|   IBIS model for TI xxx DSP
[IBIS Ver]   5.1
[Disclaimer]   Please be aware that in the absence of a written agreement
|   Texas Instruments(TI) assumes no liability for:
|   (1) The accuracy of the IBIS models provided to your company,
|   however, the IBIS model is compliant to industry standard
|   IQ Level 2a.  Refer to IBIS Quality Section below for
|   for full details.
|   (2) The proper functioning of these Models in your design
|   or for any resulting applications
|   (3) Infringement of patents, copyrights or intellectual
|   property rights resulting from your use of these
|   models.
|   TI provides IBIS Models as a service to our customers and
|   therefore reserves the right to limit distribution of the
|   Models.  The information is subject to change without notice.
[File Name]  sprm842a.ibs
[File Rev]   0.3
|   - Initial version
|   - Removed unsupported LVDS models
|   - Removed unsupported IIC and eMMC models
[Date]   19 Oct 2023
[Source]   Texas Instruments Incorporated
[Copyright]   Property of Texas Instruments Incorporated.
|   Unauthorized reproduction and/or distribution is strictly.
|   prohibited.
|   This product is protected under copyright law and trade
|   secret law as an unpublished work.
|   Created 2012,(C) Copyright 1999-2012,
|   Texas Instruments Incorporated., All Rights Reserved.
|   These commodities are under the U.S. Government
|   distribution license control. As such,they are not to be
|   re-exported without the prior approval of the U.S.
|   Department of Commerce.
[Notes]
   This file does not include AMI models for SerDes based links.
   For SerDes simulations use Texas Instruments IBIS AMI models
   Some IV curves contain Non monotonic data points.
|   Revision History
|   GERNERAL COMMENT: All IBIS Quality Notes below reflect latest release
|   and version of IBIS File
|   File passes ibischk5.1 and ibischk6 with 0 errors and 119 warnings
|   Component AM62SiP
[Component] AM62SiP
[Manufacturer] Texas Instruments
[Package]
|   typ   min   max
R_pkg   0.2912   0.11996   0.51217
L_pkg   2.14e-9   9.0745e-10   4.399e-9
C_pkg   6.002e-13   3.435e-13   1.03e-12
[Package Model]   am62sip_pkg
[Pin]	Signal_name	model_name
F6	ATEST0		NC
AE2	ATEST1		NC
AA12	CSI0_ATB_0_H	NC
Y15	CSI0_ATB_1_H	NC
AD15	CSI0_RXCLKN	NC
AE15	CSI0_RXCLKP	NC
AB14	CSI0_RXN0	NC
AD14	CSI0_RXN1	NC
AD13	CSI0_RXN2	NC
AB12	CSI0_RXN3	NC
AC15	CSI0_RXP0	NC
AE14	CSI0_RXP1	NC
AE13	CSI0_RXP2	NC
AC13	CSI0_RXP3	NC
AA14	CSI0_RXRCALIB	NC
R3	DDR_ZQ		NC
T2	DDR0_ATB0	NC
U4	DDR0_ATB1	NC
M2	DDR0_CAL0	NC
G1	DDR0_RESET0_N	NC
E12	EMU0		LVCMOS_V
C11	EMU1		LVCMOS_V
A18	EXT_REFCLK1	LVCMOS_V
D16	EXTINTN		IIC_V
M25	GPMC0_AD0	LVCMOS_H
N23	GPMC0_AD1	LVCMOS_H
T25	GPMC0_AD10	LVCMOS_H
R21	GPMC0_AD11	LVCMOS_H
T22	GPMC0_AD12	LVCMOS_H
T24	GPMC0_AD13	LVCMOS_H
U25	GPMC0_AD14	LVCMOS_H
U24	GPMC0_AD15	LVCMOS_H
N24	GPMC0_AD2	LVCMOS_H
N25	GPMC0_AD3	LVCMOS_H
P24	GPMC0_AD4	LVCMOS_H
P22	GPMC0_AD5	LVCMOS_H
P21	GPMC0_AD6	LVCMOS_H
R23	GPMC0_AD7	LVCMOS_H
R24	GPMC0_AD8	LVCMOS_H
R25	GPMC0_AD9	LVCMOS_H
L23	GPMC0_ADVN_ALE	LVCMOS_H
M24	GPMC0_BE0N_CLE	LVCMOS_H
N20	GPMC0_BE1N	LVCMOS_H
P25	GPMC0_CLK	LVCMOS_H
M21	GPMC0_CSN0	LVCMOS_H
L21	GPMC0_CSN1	LVCMOS_H
K22	GPMC0_CSN2	LVCMOS_H
K24	GPMC0_CSN3	LVCMOS_H
M22	GPMC0_DIR	LVCMOS_H
L24	GPMC0_OEN_REN	LVCMOS_H
U23	GPMC0_WAIT0	LVCMOS_H
V25	GPMC0_WAIT1	LVCMOS_H
L25	GPMC0_WEN	LVCMOS_H
K25	GPMC0_WPN	LVCMOS_H
B16	I2C0_SCL	LVCMOS_V
A16	I2C0_SDA	LVCMOS_V
B17	I2C1_SCL	LVCMOS_V
A17	I2C1_SDA	LVCMOS_V
B1	IFORCE		NC
E15	MCAN0_RX	LVCMOS_V
C15	MCAN0_TX	LVCMOS_V
A20	MCASP0_ACLKR	LVCMOS_V
B20	MCASP0_ACLKX	LVCMOS_V
E19	MCASP0_AFSR	LVCMOS_V
D20	MCASP0_AFSX	LVCMOS_V
E18	MCASP0_AXR0	LVCMOS_V
B18	MCASP0_AXR1	LVCMOS_V
A19	MCASP0_AXR2	LVCMOS_V
B19	MCASP0_AXR3	LVCMOS_V
D1	MCU_ERRORN	LVCMOS_H
A8	MCU_I2C0_SCL	IIC_V
D10	MCU_I2C0_SDA	IIC_V
B3	MCU_MCAN0_RX	LVCMOS_V
D6	MCU_MCAN0_TX	LVCMOS_V
D4	MCU_MCAN1_RX	LVCMOS_V
E5	MCU_MCAN1_TX	LVCMOS_V
B2	MCU_OSC0_XI	NC
A3	MCU_OSC0_XO	NC
D2	MCU_PORZ	RESET_H
B12	MCU_RESETSTATZ	LVCMOS_V
E11	MCU_RESETZ	LVCMOS_V
A7	MCU_SPI0_CLK	LVCMOS_V
E8	MCU_SPI0_CS0	LVCMOS_V
B8	MCU_SPI0_CS1	LVCMOS_V
D9	MCU_SPI0_D0	LVCMOS_V
C9	MCU_SPI0_D1	LVCMOS_V
A6	MCU_UART0_CTSN	LVCMOS_V
B6	MCU_UART0_RTSN	LVCMOS_V
B5	MCU_UART0_RXD	LVCMOS_V
A5	MCU_UART0_TXD	LVCMOS_V
AD24	MDIO0_MDC	LVCMOS_V
AB22	MDIO0_MDIO	LVCMOS_V
AB1	MMC0_CLK	SDIO_H
Y3	MMC0_CMD	SDIO_H
AA2	MMC0_DAT0	SDIO_H
AA1	MMC0_DAT1	SDIO_H
AA3	MMC0_DAT2	SDIO_H
Y4	MMC0_DAT3	SDIO_H
AB2	MMC0_DAT4	SDIO_H
AC1	MMC0_DAT5	SDIO_H
AD2	MMC0_DAT6	SDIO_H
AC2	MMC0_DAT7	SDIO_H
B22	MMC1_CLK	SDIO_V
A21	MMC1_CMD	SDIO_V
A22	MMC1_DAT0	SDIO_V
B21	MMC1_DAT1	SDIO_V
C21	MMC1_DAT2	SDIO_V
D22	MMC1_DAT3	SDIO_V
D17	MMC1_SDCD	LVCMOS_V
C17	MMC1_SDWP	LVCMOS_V
D25	MMC2_CLK	SDIO_H
C24	MMC2_CMD	SDIO_H
B24	MMC2_DAT0	SDIO_H
C25	MMC2_DAT1	SDIO_H
E23	MMC2_DAT2	SDIO_H
D24	MMC2_DAT3	SDIO_H
A23	MMC2_SDCD	LVCMOS_H
B23	MMC2_SDWP	LVCMOS_H
AA5	OLDI0_A0N	LVDS
Y6	OLDI0_A0P	LVDS
AD3	OLDI0_A1N	LVDS
AB4	OLDI0_A1P	LVDS
Y8	OLDI0_A2N	LVDS
AA8	OLDI0_A2P	LVDS
AB6	OLDI0_A3N	LVDS
AA7	OLDI0_A3P	LVDS
AC6	OLDI0_A4N	LVDS
AC5	OLDI0_A4P	LVDS
AE5	OLDI0_A5N	LVDS
AD6	OLDI0_A5P	LVDS
AE6	OLDI0_A6N	LVDS
AD7	OLDI0_A6P	LVDS
AD8	OLDI0_A7N	LVDS
AE7	OLDI0_A7P	LVDS
AD4	OLDI0_CLK0N	LVDS
AE3	OLDI0_CLK0P	LVDS
AE4	OLDI0_CLK1N	LVDS
AD5	OLDI0_CLK1P	LVDS
H24	OSPI0_CLK	LVCMOS_H
F23	OSPI0_CSN0	LVCMOS_H
G21	OSPI0_CSN1	LVCMOS_H
H21	OSPI0_CSN2	LVCMOS_H
E24	OSPI0_CSN3	LVCMOS_H
E25	OSPI0_D0	LVCMOS_H
G24	OSPI0_D1	LVCMOS_H
F25	OSPI0_D2	LVCMOS_H
F24	OSPI0_D3	LVCMOS_H
J23	OSPI0_D4	LVCMOS_H
J25	OSPI0_D5	LVCMOS_H
H25	OSPI0_D6	LVCMOS_H
J22	OSPI0_D7	LVCMOS_H
J24	OSPI0_DQS	LVCMOS_H
G25	OSPI0_LBCLKO	LVCMOS_H
B7	PMIC_LPM_EN0	LVCMOS_V
E21	PORZ_OUT	LVCMOS_V
F20	RESET_REQZ	LVCMOS_V
F22	RESETSTATZ	LVCMOS_V
AB17	RGMII1_RD0	LVCMOS_V
AC17	RGMII1_RD1	LVCMOS_V
AB16	RGMII1_RD2	LVCMOS_V
AA15	RGMII1_RD3	LVCMOS_V
AE17	RGMII1_RX_CTL	LVCMOS_V
AD17	RGMII1_RXC	LVCMOS_V
AE20	RGMII1_TD0	LVCMOS_V
AD20	RGMII1_TD1	LVCMOS_V
AE18	RGMII1_TD2	LVCMOS_V
AD18	RGMII1_TD3	LVCMOS_V
AD19	RGMII1_TX_CTL	LVCMOS_V
AE19	RGMII1_TXC	LVCMOS_V
AE23	RGMII2_RD0	LVCMOS_V
AB20	RGMII2_RD1	LVCMOS_V
AC21	RGMII2_RD2	LVCMOS_V
AE22	RGMII2_RD3	LVCMOS_V
AD22	RGMII2_RX_CTL	LVCMOS_V
AD23	RGMII2_RXC	LVCMOS_V
Y18	RGMII2_TD0	LVCMOS_V
AA18	RGMII2_TD1	LVCMOS_V
AD21	RGMII2_TD2	LVCMOS_V
AC20	RGMII2_TD3	LVCMOS_V
AA19	RGMII2_TX_CTL	LVCMOS_V
AE21	RGMII2_TXC	LVCMOS_V
A14	SPI0_CLK	LVCMOS_V
A13	SPI0_CS0	LVCMOS_V
C13	SPI0_CS1	LVCMOS_V
B13	SPI0_D0		LVCMOS_V
B14	SPI0_D1		LVCMOS_V
A10	TCK		LVCMOS_V
A11	TDI		LVCMOS_V
D12	TDO		LVCMOS_V
E7	TEMP_DIODE_P	NC
B11	TMS		LVCMOS_V
B10	TRSTN		LVCMOS_V
A15	UART0_CTSN	LVCMOS_V
B15	UART0_RTSN	LVCMOS_V
D14	UART0_RXD	LVCMOS_V
E14	UART0_TXD	LVCMOS_V
AE11	USB0_DM		NC
AD11	USB0_DP		NC
C20	USB0_DRVVBUS	LVCMOS_V
AE10	USB0_RCALIB	NC
AC11	USB0_VBUS	NC
AD10	USB1_DM		NC
AE9	USB1_DP		NC
F18	USB1_DRVVBUS	LVCMOS_V
AC9	USB1_RCALIB	NC
AB10	USB1_VBUS	NC
U22	VOUT0_DATA0	LVCMOS_H
V24	VOUT0_DATA1	LVCMOS_H
V20	VOUT0_DATA10	LVCMOS_H
AA23	VOUT0_DATA11	LVCMOS_H
AB25	VOUT0_DATA12	LVCMOS_H
AA24	VOUT0_DATA13	LVCMOS_H
Y22	VOUT0_DATA14	LVCMOS_H
AA21	VOUT0_DATA15	LVCMOS_H
W25	VOUT0_DATA2	LVCMOS_H
W24	VOUT0_DATA3	LVCMOS_H
Y25	VOUT0_DATA4	LVCMOS_H
Y24	VOUT0_DATA5	LVCMOS_H
Y23	VOUT0_DATA6	LVCMOS_H
AA25	VOUT0_DATA7	LVCMOS_H
V21	VOUT0_DATA8	LVCMOS_H
W21	VOUT0_DATA9	LVCMOS_H
Y20	VOUT0_DE	LVCMOS_H
AB24	VOUT0_HSYNC	LVCMOS_H
AC24	VOUT0_PCLK	LVCMOS_H
AC25	VOUT0_VSYNC	LVCMOS_H
A2	VSENSE		NC
A12	WKUP_CLKOUT0	LVCMOS_V
B9	WKUP_I2C0_SCL	IIC_V
A9	WKUP_I2C0_SDA	IIC_V
C2	WKUP_LFOSC0_XI	NC
C1	WKUP_LFOSC0_XO	NC
C6	WKUP_UART0_CTSN	LVCMOS_V
A4	WKUP_UART0_RTSN	LVCMOS_V
B4	WKUP_UART0_RXD	LVCMOS_V
C5	WKUP_UART0_TXD	LVCMOS_V
A1	VSS	GND
A24	VSS	GND
A25	VSS	GND
B25	VSS	GND
E1	VSS	GND
E2	VSS	GND
E3	VSS	GND
F1	VSS	GND
F3	VSS	GND
F4	VSS	GND
F13	VSS	GND
G5	VSS	GND
G13	VSS	GND
G19	VSS	GND
H5	VSS	GND
H6	VSS	GND
H13	VSS	GND
H16	VSS	GND
H18	VSS	GND
H20	VSS	GND
J1	VSS	GND
J2	VSS	GND
J3	VSS	GND
J4	VSS	GND
J7	VSS	GND
J13	VSS	GND
K1	VSS	GND
K2	VSS	GND
K3	VSS	GND
K4	VSS	GND
K7	VSS	GND
K13	VSS	GND
K15	VSS	GND
K19	VSS	GND
L1	VSS	GND
L2	VSS	GND
L5	VSS	GND
L6	VSS	GND
L20	VSS	GND
M1	VSS	GND
M5	VSS	GND
M7	VSS	GND
M8	VSS	GND
M10	VSS	GND
M12	VSS	GND
M13	VSS	GND
M17	VSS	GND
M18	VSS	GND
N6	VSS	GND
N15	VSS	GND
P1	VSS	GND
P4	VSS	GND
P5	VSS	GND
P7	VSS	GND
P10	VSS	GND
P13	VSS	GND
R1	VSS	GND
R5	VSS	GND
R6	VSS	GND
R13	VSS	GND
R15	VSS	GND
R18	VSS	GND
R20	VSS	GND
T1	VSS	GND
T4	VSS	GND
T8	VSS	GND
T13	VSS	GND
T14	VSS	GND
T16	VSS	GND
T17	VSS	GND
T18	VSS	GND
U3	VSS	GND
U8	VSS	GND
U19	VSS	GND
V1	VSS	GND
V5	VSS	GND
V6	VSS	GND
V9	VSS	GND
V10	VSS	GND
V11	VSS	GND
V13	VSS	GND
V16	VSS	GND
V18	VSS	GND
W1	VSS	GND
W5	VSS	GND
W7	VSS	GND
Y1	VSS	GND
Y2	VSS	GND
AA11	VSS	GND
AB9	VSS	GND
AD1	VSS	GND
AD9	VSS	GND
AD12	VSS	GND
AD16	VSS	GND
AD25	VSS	GND
AE1	VSS	GND
AE8	VSS	GND
AE12	VSS	GND
AE16	VSS	GND
AE24	VSS	GND
AE25	VSS	GND
G9	CAP_VDDS_CANUART	POWER
H11	CAP_VDDS_MCU	POWER
H15	CAP_VDDS0	POWER
K18	CAP_VDDS1	POWER
W17	CAP_VDDS2	POWER
P19	CAP_VDDS3	POWER
U7	CAP_VDDS4	POWER
H17	CAP_VDDS5	POWER
J19	CAP_VDDS6	POWER
F8	VDD_CANUART	POWER
H8	VDD_CORE	POWER
J11	VDD_CORE	POWER
J14	VDD_CORE	POWER
K17	VDD_CORE	POWER
L12	VDD_CORE	POWER
L15	VDD_CORE	POWER
M16	VDD_CORE	POWER
N8	VDD_CORE	POWER
N11	VDD_CORE	POWER
N13	VDD_CORE	POWER
P17	VDD_CORE	POWER
R11	VDD_CORE	POWER
R14	VDD_CORE	POWER
U12	VDD_CORE	POWER
V8	VDD_CORE	POWER
V15	VDD_CORE	POWER
V17	VDD_CORE	POWER
W14	VDDA_1P8_CSIRX0	POWER
W9	VDDA_1P8_OLDI0	POWER
W10	VDDA_1P8_OLDI0	POWER
Y11	VDDA_1P8_USB	POWER
Y13	VDDA_3P3_USB	POWER
W13	VDDA_CORE_CSIRX0	POWER
W12	VDDA_CORE_USB	POWER
L11	VDDA_MCU	POWER
U11	VDDA_PLL0	POWER
U15	VDDA_PLL1	POWER
L14	VDDA_PLL2	POWER
T9	VDDA_TEMP0	POWER
G16	VDDA_TEMP1	POWER
J12	VDDR_CORE	POWER
K16	VDDR_CORE	POWER
N12	VDDR_CORE	POWER
N14	VDDR_CORE	POWER
P16	VDDR_CORE	POWER
R12	VDDR_CORE	POWER
T10	VDDR_CORE	POWER
U14	VDDR_CORE	POWER
K9	VDDS_DDR	POWER
L8	VDDS_DDR	POWER
M9	VDDS_DDR	POWER
P9	VDDS_DDR	POWER
R8	VDDS_DDR	POWER
F2	VDDS_DDR_MEM	POWER
G2	VDDS_DDR_MEM	POWER
H1	VDDS_DDR_MEM	POWER
H2	VDDS_DDR_MEM	POWER
N1	VDDS_DDR_MEM	POWER
N2	VDDS_DDR_MEM	POWER
P2	VDDS_DDR_MEM	POWER
R2	VDDS_DDR_MEM	POWER
U1	VDDS_DDR_MEM	POWER
U2	VDDS_DDR_MEM	POWER
V2	VDDS_DDR_MEM	POWER
W2	VDDS_DDR_MEM	POWER
M4	VDDS_MEM_1P8	POWER
N3	VDDS_MEM_1P8	POWER
G7	VDDS_OSC0	POWER
H9	VDDSHV_CANUART	POWER
F11	VDDSHV_MCU	POWER
G12	VDDSHV_MCU	POWER
F15	VDDSHV0		POWER
G14	VDDSHV0		POWER
L18	VDDSHV1		POWER
M19	VDDSHV1		POWER
W16	VDDSHV2		POWER
W19	VDDSHV2		POWER
N18	VDDSHV3		POWER
P18	VDDSHV3		POWER
T19	VDDSHV3		POWER
U18	VDDSHV3		POWER
T7	VDDSHV4		POWER
G17	VDDSHV5		POWER
J18	VDDSHV6		POWER
G10	VMON_1P8_SOC	POWER
K10	VMON_3P3_SOC	POWER
H10	VMON_ER_VSYS	POWER
J8	VPP		POWER
|********************  DIFF PIN  *******************************
[Diff_pin]   inv_pin vdiff tdelay_typ   tdelay_min  tdelay_max
AA5	Y6	NA	NA	NA	NA	||	OLDI0_A0N	&	OLDI0_A0P
AD3	AB4	NA	NA	NA	NA	||	OLDI0_A1N	&	OLDI0_A1P
Y8	AA8	NA	NA	NA	NA	||	OLDI0_A2N	&	OLDI0_A2P
AB6	AA7	NA	NA	NA	NA	||	OLDI0_A3N	&	OLDI0_A3P
AC6	AC5	NA	NA	NA	NA	||	OLDI0_A4N	&	OLDI0_A4P
AE5	AD6	NA	NA	NA	NA	||	OLDI0_A5N	&	OLDI0_A5P
AE6	AD7	NA	NA	NA	NA	||	OLDI0_A6N	&	OLDI0_A6P
AD8	AE7	NA	NA	NA	NA	||	OLDI0_A7N	&	OLDI0_A7P
AD4	AE3	NA	NA	NA	NA	||	OLDI0_CLK0N	&	OLDI0_CLK0P
AE4	AD5	NA	NA	NA	NA	||	OLDI0_CLK1N	&	OLDI0_CLK1P
|****************** SDIO
[Model Selector] SDIO_H
sdio1_r40_1p8_h PRWDWUWSWEWCDGSDIO_H@_R40_1p8_comment
sdio1_r40_3p3_h PRWDWUWSWEWCDGSDIO_H@_R40_3p3_comment
[Model Selector] SDIO_V
sdio0_r40_1p8_v PRWDWUWSWEWCDGSDIO_V@_R40_1p8_comment
sdio0_r40_3p3_v PRWDWUWSWEWCDGSDIO_V@_R40_3p3_comment
|********** LVCMOS
[Model Selector] LVCMOS_H
lvcmos1_nom_1p8_h PRWDWUWSWEWCDGLVCMOS_H@_Nom_1p8_comment
lvcmos1_nom_3p3_h PRWDWUWSWEWCDGLVCMOS_H@_Nom_3p3_comment
[Model Selector] LVCMOS_V
lvcmos0_nom_1p8_v PRWDWUWSWEWCDGLVCMOS_V@_Nom_1p8_comment
lvcmos0_nom_3p3_v PRWDWUWSWEWCDGLVCMOS_V@_Nom_3p3_comment
[Model Selector] IIC_V
IIC18_1_0_V PRBOPDDGZIIC_V@HSMODE_HSMCSE=0_0_comment 1.8V
IIC18_1_1_V PRBOPDDGZIIC_V@HSMODE_HSMCSE=0_1_comment 1.8V
IIC18_1_2_V PRBOPDDGZIIC_V@HSMODE_HSMCSE=1_0_comment 1.8V
IIC18_1_3_V PRBOPDDGZIIC_V@HSMODE_HSMCSE=1_1_comment 1.8V
IIC33_1_0_V PRBOPDDGZIIC_V@HSMODE_HSMCSE=0_0_comment
[Model Selector] LVDS
lvds_tx_03   LVDS TX Driver Permumentation 03
lvds_tx_11   LVDS TX Driver Permumentation 11
|***************** RESET ************************************************
[Model Selector] RESET_H
reset18_0_0 PDIDGZRESET_H
|   EMMC
[MODEL SELECTOR] EMMC
emmc51_io_tx40ohm   40ohm DRIVER
|   Package Model
[Define Package Model]   am62sip_pkg
[Manufacturer]   Name1
[OEM]   Name2
[Description]   275-pin Package
|[Number of Sections]   1
[Number of Pins]   275
[Pin Numbers]
|[Pin Name]  Net Number   Net Name   Net's All Pins
H15   | 1   CAP_VDDS0   H15
K18   | 2   CAP_VDDS1   K18
W17   | 3   CAP_VDDS2   W17
P19   | 4   CAP_VDDS3   P19
U7   | 5   CAP_VDDS4   U7
H17   | 6   CAP_VDDS5   H17
J19   | 7   CAP_VDDS6   J19
G9   | 8   CAP_VDDS_CANUART   G9
H11   | 9   CAP_VDDS_MCU   H11
W14   | 10   VDDA_1P8_CSIRX0   W14
W9   | 11   VDDA_1P8_OLDI0   W9
   |W10
Y11   | 12   VDDA_1P8_USB   Y11
Y13   | 13   VDDA_3P3_USB   Y13
W13   | 14   VDDA_CORE_CSIRX0   W13
W12   | 15   VDDA_CORE_USB   W12
L11   | 16   VDDA_MCU   L11
U11   | 17   VDDA_PLL0   U11
U15   | 18   VDDA_PLL1   U15
L14   | 19   VDDA_PLL2   L14
T9   | 20   VDDA_TEMP0   T9
G16   | 21   VDDA_TEMP1   G16
J12   | 22   VDDR_CORE   J12
   |K16
   |N12
   |N14
   |P16
   |R12
   |T10
   |U14
F15   | 23   VDDSHV0   F15
   |G14
L18   | 24   VDDSHV1   L18
   |M19
W16   | 25   VDDSHV2   W16
   |W19
N18   | 26   VDDSHV3   N18
   |P18
   |T19
   |U18
T7   | 27   VDDSHV4   T7
G17   | 28   VDDSHV5   G17
J18   | 29   VDDSHV6   J18
H9   | 30   VDDSHV_CANUART   H9
F11   | 31   VDDSHV_MCU   F11
   |G12
K9   | 32   VDDS_DDR   K9
   |L8
   |M9
   |P9
   |R8
G7   | 33   VDDS_OSC0   G7
F8   | 34   VDD_CANUART   F8
H8   | 35   VDD_CORE   H8
   |J11
   |J14
   |K17
   |L12
   |L15
   |M16
   |N8
   |N11
   |N13
   |P17
   |R11
   |R14
   |U12
   |V8
   |V15
   |V17
F6   | 36   ATEST0   F6
AE2   | 37   ATEST1   AE2
AA12   | 38   CSI0_ATB_0_H   AA12
Y15   | 39   CSI0_ATB_1_H   Y15
AD15   | 40   CSI0_RXCLKN   AD15
AE15   | 41   CSI0_RXCLKP   AE15
AB14   | 42   CSI0_RXN0   AB14
AD14   | 43   CSI0_RXN1   AD14
AD13   | 44   CSI0_RXN2   AD13
AB12   | 45   CSI0_RXN3   AB12
AC15   | 46   CSI0_RXP0   AC15
AE14   | 47   CSI0_RXP1   AE14
AE13   | 48   CSI0_RXP2   AE13
AC13   | 49   CSI0_RXP3   AC13
AA14   | 50   CSI0_RXRCALIB   AA14
T2   | 51   DDR0_ATB0   T2
U4   | 52   DDR0_ATB1   U4
M2   | 53   DDR0_CAL0   M2
G1   | 54   DDR0_RESET0_N   G1
R3   | 55   DDR_ZQ   R3
E12   | 56   EMU0   E12
C11   | 57   EMU1   C11
D16   | 58   EXTINTN   D16
A18   | 59   EXT_REFCLK1   A18
M25   | 60   GPMC0_AD0   M25
N23   | 61   GPMC0_AD1   N23
N24   | 62   GPMC0_AD2   N24
N25   | 63   GPMC0_AD3   N25
P24   | 64   GPMC0_AD4   P24
P22   | 65   GPMC0_AD5   P22
P21   | 66   GPMC0_AD6   P21
R23   | 67   GPMC0_AD7   R23
R24   | 68   GPMC0_AD8   R24
R25   | 69   GPMC0_AD9   R25
T25   | 70   GPMC0_AD10   T25
R21   | 71   GPMC0_AD11   R21
T22   | 72   GPMC0_AD12   T22
T24   | 73   GPMC0_AD13   T24
U25   | 74   GPMC0_AD14   U25
U24   | 75   GPMC0_AD15   U24
L23   | 76   GPMC0_ADVN_ALE   L23
M24   | 77   GPMC0_BE0N_CLE   M24
N20   | 78   GPMC0_BE1N   N20
P25   | 79   GPMC0_CLK   P25
M21   | 80   GPMC0_CSN0   M21
L21   | 81   GPMC0_CSN1   L21
K22   | 82   GPMC0_CSN2   K22
K24   | 83   GPMC0_CSN3   K24
M22   | 84   GPMC0_DIR   M22
L24   | 85   GPMC0_OEN_REN   L24
U23   | 86   GPMC0_WAIT0   U23
V25   | 87   GPMC0_WAIT1   V25
L25   | 88   GPMC0_WEN   L25
K25   | 89   GPMC0_WPN   K25
B16   | 90   I2C0_SCL   B16
A16   | 91   I2C0_SDA   A16
B17   | 92   I2C1_SCL   B17
A17   | 93   I2C1_SDA   A17
B1   | 94   IFORCE   B1
E15   | 95   MCAN0_RX   E15
C15   | 96   MCAN0_TX   C15
A20   | 97   MCASP0_ACLKR   A20
B20   | 98   MCASP0_ACLKX   B20
E19   | 99   MCASP0_AFSR   E19
D20   | 100   MCASP0_AFSX   D20
E18   | 101   MCASP0_AXR0   E18
B18   | 102   MCASP0_AXR1   B18
A19   | 103   MCASP0_AXR2   A19
B19   | 104   MCASP0_AXR3   B19
D1   | 105   MCU_ERRORN   D1
A8   | 106   MCU_I2C0_SCL   A8
D10   | 107   MCU_I2C0_SDA   D10
B3   | 108   MCU_MCAN0_RX   B3
D6   | 109   MCU_MCAN0_TX   D6
D4   | 110   MCU_MCAN1_RX   D4
E5   | 111   MCU_MCAN1_TX   E5
B2   | 112   MCU_OSC0_XI   B2
A3   | 113   MCU_OSC0_XO   A3
D2   | 114   MCU_PORZ   D2
B12   | 115   MCU_RESETSTATZ   B12
E11   | 116   MCU_RESETZ   E11
A7   | 117   MCU_SPI0_CLK   A7
E8   | 118   MCU_SPI0_CS0   E8
B8   | 119   MCU_SPI0_CS1   B8
D9   | 120   MCU_SPI0_D0   D9
C9   | 121   MCU_SPI0_D1   C9
A6   | 122   MCU_UART0_CTSN   A6
B6   | 123   MCU_UART0_RTSN   B6
B5   | 124   MCU_UART0_RXD   B5
A5   | 125   MCU_UART0_TXD   A5
AD24   | 126   MDIO0_MDC   AD24
AB22   | 127   MDIO0_MDIO   AB22
AB1   | 128   MMC0_CLK   AB1
Y3   | 129   MMC0_CMD   Y3
AA2   | 130   MMC0_DAT0   AA2
AA1   | 131   MMC0_DAT1   AA1
AA3   | 132   MMC0_DAT2   AA3
Y4   | 133   MMC0_DAT3   Y4
AB2   | 134   MMC0_DAT4   AB2
AC1   | 135   MMC0_DAT5   AC1
AD2   | 136   MMC0_DAT6   AD2
AC2   | 137   MMC0_DAT7   AC2
B22   | 138   MMC1_CLK   B22
A21   | 139   MMC1_CMD   A21
A22   | 140   MMC1_DAT0   A22
B21   | 141   MMC1_DAT1   B21
C21   | 142   MMC1_DAT2   C21
D22   | 143   MMC1_DAT3   D22
D17   | 144   MMC1_SDCD   D17
C17   | 145   MMC1_SDWP   C17
D25   | 146   MMC2_CLK   D25
C24   | 147   MMC2_CMD   C24
B24   | 148   MMC2_DAT0   B24
C25   | 149   MMC2_DAT1   C25
E23   | 150   MMC2_DAT2   E23
D24   | 151   MMC2_DAT3   D24
A23   | 152   MMC2_SDCD   A23
B23   | 153   MMC2_SDWP   B23
AA5   | 154   OLDI0_A0N   AA5
Y6   | 155   OLDI0_A0P   Y6
AD3   | 156   OLDI0_A1N   AD3
AB4   | 157   OLDI0_A1P   AB4
Y8   | 158   OLDI0_A2N   Y8
AA8   | 159   OLDI0_A2P   AA8
AB6   | 160   OLDI0_A3N   AB6
AA7   | 161   OLDI0_A3P   AA7
AC6   | 162   OLDI0_A4N   AC6
AC5   | 163   OLDI0_A4P   AC5
AE5   | 164   OLDI0_A5N   AE5
AD6   | 165   OLDI0_A5P   AD6
AE6   | 166   OLDI0_A6N   AE6
AD7   | 167   OLDI0_A6P   AD7
AD8   | 168   OLDI0_A7N   AD8
AE7   | 169   OLDI0_A7P   AE7
AD4   | 170   OLDI0_CLK0N   AD4
AE3   | 171   OLDI0_CLK0P   AE3
AE4   | 172   OLDI0_CLK1N   AE4
AD5   | 173   OLDI0_CLK1P   AD5
H24   | 174   OSPI0_CLK   H24
F23   | 175   OSPI0_CSN0   F23
G21   | 176   OSPI0_CSN1   G21
H21   | 177   OSPI0_CSN2   H21
E24   | 178   OSPI0_CSN3   E24
E25   | 179   OSPI0_D0   E25
G24   | 180   OSPI0_D1   G24
F25   | 181   OSPI0_D2   F25
F24   | 182   OSPI0_D3   F24
J23   | 183   OSPI0_D4   J23
J25   | 184   OSPI0_D5   J25
H25   | 185   OSPI0_D6   H25
J22   | 186   OSPI0_D7   J22
J24   | 187   OSPI0_DQS   J24
G25   | 188   OSPI0_LBCLKO   G25
B7   | 189   PMIC_LPM_EN0   B7
E21   | 190   PORZ_OUT   E21
F22   | 191   RESETSTATZ   F22
F20   | 192   RESET_REQZ   F20
AB17   | 193   RGMII1_RD0   AB17
AC17   | 194   RGMII1_RD1   AC17
AB16   | 195   RGMII1_RD2   AB16
AA15   | 196   RGMII1_RD3   AA15
AD17   | 197   RGMII1_RXC   AD17
AE17   | 198   RGMII1_RX_CTL   AE17
AE20   | 199   RGMII1_TD0   AE20
AD20   | 200   RGMII1_TD1   AD20
AE18   | 201   RGMII1_TD2   AE18
AD18   | 202   RGMII1_TD3   AD18
AE19   | 203   RGMII1_TXC   AE19
AD19   | 204   RGMII1_TX_CTL   AD19
AE23   | 205   RGMII2_RD0   AE23
AB20   | 206   RGMII2_RD1   AB20
AC21   | 207   RGMII2_RD2   AC21
AE22   | 208   RGMII2_RD3   AE22
AD23   | 209   RGMII2_RXC   AD23
AD22   | 210   RGMII2_RX_CTL   AD22
Y18   | 211   RGMII2_TD0   Y18
AA18   | 212   RGMII2_TD1   AA18
AD21   | 213   RGMII2_TD2   AD21
AC20   | 214   RGMII2_TD3   AC20
AE21   | 215   RGMII2_TXC   AE21
AA19   | 216   RGMII2_TX_CTL   AA19
A14   | 217   SPI0_CLK   A14
A13   | 218   SPI0_CS0   A13
C13   | 219   SPI0_CS1   C13
B13   | 220   SPI0_D0   B13
B14   | 221   SPI0_D1   B14
A10   | 222   TCK   A10
A11   | 223   TDI   A11
D12   | 224   TDO   D12
E7   | 225   TEMP_DIODE_P   E7
B11   | 226   TMS   B11
B10   | 227   TRSTN   B10
A15   | 228   UART0_CTSN   A15
B15   | 229   UART0_RTSN   B15
D14   | 230   UART0_RXD   D14
E14   | 231   UART0_TXD   E14
AE11   | 232   USB0_DM   AE11
AD11   | 233   USB0_DP   AD11
C20   | 234   USB0_DRVVBUS   C20
AE10   | 235   USB0_RCALIB   AE10
AC11   | 236   USB0_VBUS   AC11
AD10   | 237   USB1_DM   AD10
AE9   | 238   USB1_DP   AE9
F18   | 239   USB1_DRVVBUS   F18
AC9   | 240   USB1_RCALIB   AC9
AB10   | 241   USB1_VBUS   AB10
G10   | 242   VMON_1P8_SOC   G10
K10   | 243   VMON_3P3_SOC   K10
H10   | 244   VMON_ER_VSYS   H10
U22   | 245   VOUT0_DATA0   U22
V24   | 246   VOUT0_DATA1   V24
W25   | 247   VOUT0_DATA2   W25
W24   | 248   VOUT0_DATA3   W24
Y25   | 249   VOUT0_DATA4   Y25
Y24   | 250   VOUT0_DATA5   Y24
Y23   | 251   VOUT0_DATA6   Y23
AA25   | 252   VOUT0_DATA7   AA25
V21   | 253   VOUT0_DATA8   V21
W21   | 254   VOUT0_DATA9   W21
V20   | 255   VOUT0_DATA10   V20
AA23   | 256   VOUT0_DATA11   AA23
AB25   | 257   VOUT0_DATA12   AB25
AA24   | 258   VOUT0_DATA13   AA24
Y22   | 259   VOUT0_DATA14   Y22
AA21   | 260   VOUT0_DATA15   AA21
Y20   | 261   VOUT0_DE   Y20
AB24   | 262   VOUT0_HSYNC   AB24
AC24   | 263   VOUT0_PCLK   AC24
AC25   | 264   VOUT0_VSYNC   AC25
J8   | 265   VPP   J8
A2   | 266   VSENSE   A2
A12   | 267   WKUP_CLKOUT0   A12
B9   | 268   WKUP_I2C0_SCL   B9
A9   | 269   WKUP_I2C0_SDA   A9
C2   | 270   WKUP_LFOSC0_XI   C2
C1   | 271   WKUP_LFOSC0_XO   C1
C6   | 272   WKUP_UART0_CTSN   C6
A4   | 273   WKUP_UART0_RTSN   A4
B4   | 274   WKUP_UART0_RXD   B4
C5   | 275   WKUP_UART0_TXD   C5
[Model Data]
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[End Model Data]
[End Package Model]
| Models and submodels in the file (137): lvcmos1_nom_1p8_h (I/O), lvcmos0_nom_1p8_v (I/O), lvcmos1_nom_3p3_h (I/O), lvcmos0_nom_3p3_v (I/O), sdio1_r40_1p8_h (I/O), sdio0_r40_1p8_v (I/O), sdio1_r40_3p3_h (I/O), sdio0_r40_3p3_v (I/O), lpddr4_odt_120 (Input), lpddr4_odt_120_diff (Input), lpddr4_ocd_120p_120n (I/O), lpddr4_ocd_240p_240n (I/O), lpddr4_odt_240 (Input), lpddr4_ocd_40p_40n (I/O), lpddr4_odt_40 (Input), lpddr4_ocd_48p_48n (I/O), lpddr4_odt_48 (Input), lpddr4_ocd_60p_60n (I/O), lpddr4_odt_60 (Input), lpddr4_ocd_80p_80n (I/O), lpddr4_odt_80 (Input), lpddr4_odt_off (Input), lpddr4_ocd_120pd_60p_40n (I/O), lpddr4_ocd_120p_120n_diff (I/O), lpddr4_ocd_240p_240n_diff (I/O), lpddr4_odt_240_diff (Input), lpddr4_ocd_40p_40n_diff (I/O), lpddr4_odt_40_diff (Input), lpddr4_ocd_48p_48n_diff (I/O), lpddr4_odt_48_diff (Input), lpddr4_ocd_60p_60n_diff (I/O), lpddr4_odt_60_diff (Input), lpddr4_ocd_80p_80n_diff (I/O), lpddr4_ocd_120pd_60p_40n_diff (I/O), lpddr4_odt_80_diff (Input), lpddr4_odt_off_diff (Input), lpddr4_ocd_120pd_48p_40n (I/O), lpddr4_ocd_120pd_48p_40n_diff (I/O), ddr4_ocd_34p_34n (I/O), ddr4_ocd_40p_40n (I/O), ddr4_ocd_48p_48n (I/O), ddr4_ocd_60p_60n (I/O), ddr4_ocd_80p_80n (I/O), ddr4_ocd_34p_34n_diff (I/O), ddr4_ocd_40p_40n_diff (I/O), ddr4_ocd_48p_48n_diff (I/O), ddr4_ocd_60p_60n_diff (I/O), ddr4_ocd_80p_80n_diff (I/O), ddr4_odt_34 (Input), ddr4_odt_40 (Input), ddr4_odt_48 (Input), ddr4_odt_60 (Input), ddr4_odt_80 (Input), ddr4_odt_120 (Input), ddr4_odt_240 (Input), ddr4_odt_off (Input), ddr4_odt_34_diff (Input), ddr4_odt_40_diff (Input), ddr4_odt_48_diff (Input), ddr4_odt_60_diff (Input), ddr4_odt_80_diff (Input), ddr4_odt_120_diff (Input), ddr4_odt_240_diff (Input), ddr4_odt_off_diff (Input), lp4x_ocd_40p_40n (I/O), lp4x_ocd_120p_120n (I/O), lp4x_ocd_48p_48n (I/O), lp4x_ocd_34p_34n (I/O), lp4x_ocd_80p_80n (I/O), lp4x_ocd_240p_240n (I/O), lp4x_ocd_60p_60n (I/O), lp4x_0p6_ocd_80p_80n (I/O), lp4x_0p6_ocd_40p_40n (I/O), lp4x_odt_120 (Input), lp4x_odt_40 (Input), lp4x_odt_48 (Input), lp4x_odt_60 (Input), lp4x_odt_80 (Input), lp4x_odt_off (Input), lp4x_ocd_40p_40n_diff (I/O)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
